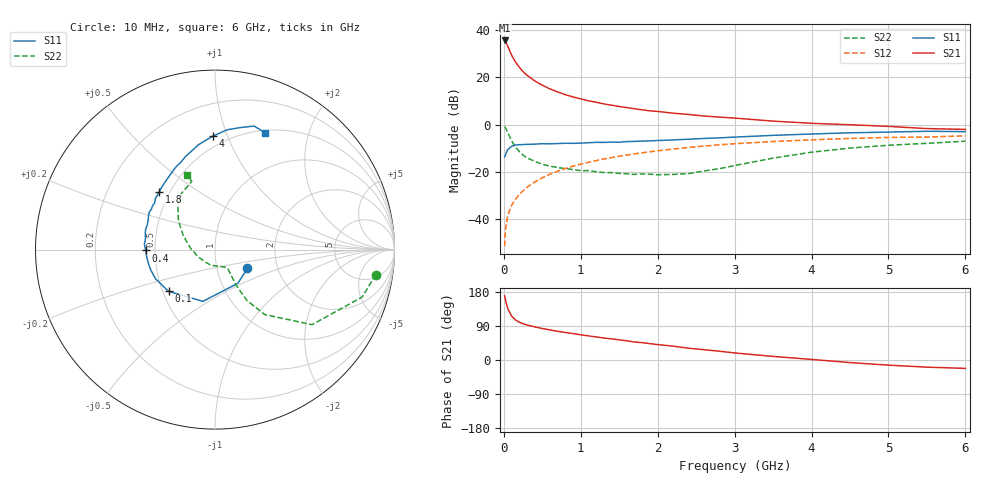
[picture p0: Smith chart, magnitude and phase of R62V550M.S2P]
! SIEMENS Small Signal Semiconductors
! BFR193
! Si NPN RF Bipolar Junction Transistor in SOT23
! VCE = 2.5 V  IC = 50 mA
! Common Emitter S-Parameters:  May  1996
# GHz  S  MA  R  50
!  f  S11  S21  S12  S22
! GHz  MAG  ANG  MAG  ANG  MAG  ANG  MAG  ANG
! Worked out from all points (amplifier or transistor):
!   36 points, 10 MHz to 6 GHz, reference 50 ohm
!   highest |S21| = 35.5 dB at 10 MHz (marker M1)
!   |S21| within 3 dB of that: start of sweep to 58.08 MHz
!   unconditionally stable (mu >= 1): 351.5 MHz to 1.96 GHz
!   at 250 MHz: K = 0.97, MSG = 25.2 dB, |S12| = -28.0 dB
!   at 1.4 GHz: K = 1.02, MAG = 10.3 dB, |S12| = -13.9 dB
!   at 6 GHz: K = 0.96, MSG = 1.4 dB, |S12| = -4.8 dB
!   S11 on the Smith chart (normalised r, x): 10 MHz: 1.40, -0.31; 100 MHz: 0.54, -0.28; 400 MHz: 0.44, -0.00; 1.8 GHz: 0.44, +0.36; 4 GHz: 0.42, +0.89; 6 GHz: 0.53, +1.38
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0.01  0.2087 -29.9  59.85 169.3  0.0027 81.9  0.9071 -8.8
0.02  0.2267 -55.7  57.19 159.3  0.0058 82.0  0.861 -17.9
0.05  0.2961 -103.1  45.42 136.4  0.0119 69.8  0.6836 -37.7
0.1  0.348 -138.1  29.53 116.3  0.0196 68.2  0.4567 -52.5
0.15  0.3685 -153.7  21.12 105.9  0.0263 70.3  0.3362 -57.8
0.2  0.3753 -161.8  16.33 99.9  0.0332 72.7  0.2703 -58.7
0.25  0.3785 -167.8  13.16 95.7  0.04 73.9  0.2267 -59.3
0.3  0.3816 -172.5  11.07 92.5  0.0471 74.6  0.1983 -58.6
0.4  0.3864 -179.3  8.412 87.5  0.0612 74.7  0.1675 -57.9
0.5  0.3947 175.4  6.78 83.1  0.0752 74.5  0.1449 -57.2
0.6  0.3919 171.3  5.66 79.5  0.0895 73.5  0.1325 -55.9
0.7  0.3982 167.1  4.887 75.6  0.1035 72.8  0.1238 -58.3
0.9  0.4017 160.3  3.834 69.8  0.1321 70.4  0.1122 -60.5
1.1  0.4136 153.8  3.176 63.7  0.1598 67.8  0.1067 -66.3
1.3  0.4202 147.4  2.734 58.0  0.1879 65.0  0.097 -72.9
1.8  0.4476 133.8  2.048 45.8  0.2538 57.4  0.0907 -97.1
2.2  0.4734 124.6  1.739 36.5  0.3046 51.2  0.0885 -128.0
3.5  0.5923 98.8  1.184 9.5  0.4386 30.4  0.1953 155.6
4  0.6319 91.1  1.064 1.5  0.4762 23.3  0.2612 141.4
4.5  0.6707 84.3  0.993 -6.8  0.5098 16.2  0.3188 130.4
5.5  0.7219 72.4  0.822 -18.9  0.5443 2.4  0.4015 108.8
6  0.7086 66.9  0.792 -22.1  0.5784 -1.6  0.4458 110.7
